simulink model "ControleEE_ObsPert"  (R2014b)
settings: Solver=ode45  StartTime=0.0  StopTime=60  RelTol=1e-6
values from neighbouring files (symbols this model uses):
  K = acker(A,B,[p p])    [para2nl.m]    (also in para2nl_PI.m = acker(Aa,Ba,[p,p,p]); PrPara2nl_PI.m = acker(Aa,Ba,[p,p,p]); TestesEE.m = acker(A,B,[p,-.6-1.02i,-.6+1.02i]); TestesEEobsPert.m = acker(A,B,[p,-.6-1.0198i,-.6+1.0198i]))
  L = L'    [para2nl.m]    (also in para2nl_PI.m; PrPara2nl_PI.m; TestesEE.m; TestesEEcanalI.m)
  Lc = L(4)    [TestesEEobsPert.m]
  Ls1 = L(5)    [TestesEEobsPert.m]
  Ls2 = L(6)    [TestesEEobsPert.m]
  Nb = gf.den{1}(1,3)/gf.num{1}(1,3)    [para2nl.m]    (also in PrPara2nl_PI.m; TestesEE.m = gf.den{1}(1,4)/gf.num{1}(1,4); TestesEEcanalI.m = -Ki/(100*p); TestesEEobsPert.m = gf.den{1}(1,4)/gf.num{1}(1,4))
  w0 = .5    (= 0.5)    [TestesEEobsPert.m]

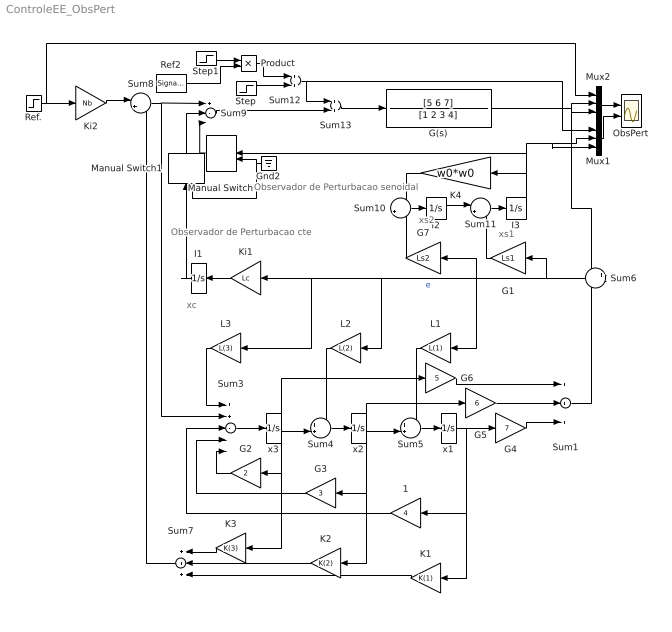
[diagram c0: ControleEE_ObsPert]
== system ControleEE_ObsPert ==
  note: xc
  note: xs1
  note: xs2
  note: Observador de Perturbacao cte
  note: Observador de Perturbacao senoidal
  1 : Gain  Gain=4
  G(s) : TransferFcn  Numerator=[5 6 7]  Denominator=[1 2 3 4]
  G1 : Gain  Gain=Ls1
  G2 : Gain  Gain=2
  G3 : Gain  Gain=3
  G4 : Gain  Gain=7
  G5 : Gain  Gain=6
  G6 : Gain  Gain=5
  G7 : Gain  Gain=Ls2
  Gnd2 : Ground
  I1 : Integrator
  I2 : Integrator
  I3 : Integrator
  K1 : Gain  Gain=K(1)
  K2 : Gain  Gain=K(2)
  K3 : Gain  Gain=K(3)
  K4 : Gain  Gain=w0*w0
  Ki1 : Gain  Gain=Lc
  Ki2 : Gain  Gain=Nb
  L1 : Gain  Gain=L(1)
  L2 : Gain  Gain=L(2)
  L3 : Gain  Gain=L(3)
  Manual Switch : ManualSwitch
  Manual Switch1 : ManualSwitch
  Mux1 : Mux  Inputs=3
  Mux2 : Mux  Inputs=3
  ObsPert : Scope  NumInputPorts=2
  Product : Product
  Ref. : Step  Time=0  SampleTime=0
  Ref2 : SignalGenerator  Amplitude=20  Frequency=w0  Units=rad/sec
  Step : Step  Time=3  After=3  SampleTime=0
  Step1 : Step  Time=2*pi/w0  SampleTime=0
  Sum1 : Sum  Inputs=+++
  Sum10 : Sum  Inputs=-+
  Sum11 : Sum  Inputs=|++
  Sum12 : Sum
  Sum13 : Sum
  Sum3 : Sum  Inputs=++---
  Sum4 : Sum  Inputs=++|
  Sum5 : Sum  Inputs=++|
  Sum6 : Sum  Inputs=+-
  Sum7 : Sum  Inputs=+++
  Sum8 : Sum  Inputs=|+-
  Sum9 : Sum  Inputs=+--
  x1 : Integrator
  x2 : Integrator
  x3 : Integrator
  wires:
  Ref./1 -> Mux2/1, Ki2/1
  Mux2/1 -> ObsPert/1
  x3/1 -> G6/1, Sum4/2, G2/1, K3/1
  x2/1 -> G5/1, Sum5/2, G3/1, K2/1
  Sum3/1 -> x3/1
  G2/1 -> Sum3/5
  G3/1 -> Sum3/4
  x1/1 -> G4/1, 1/1, K1/1
  1/1 -> Sum3/3
  G4/1 -> Sum1/3
  G5/1 -> Sum1/2
  G6/1 -> Sum1/1
  G(s)/1 -> Mux2/3, Sum6/1, Mux2/2
  Sum1/1 -> Sum6/2
  Sum13/1 -> G(s)/1
  Sum4/1 -> x2/1
  Sum5/1 -> x1/1
  Sum6/1 -> G1/1, L1/1, L2/1, L3/1, Ki1/1, G7/1  "e"
  L3/1 -> Sum3/1
  L2/1 -> Sum4/1
  L1/1 -> Sum5/1
  K3/1 -> Sum7/1
  K2/1 -> Sum7/2
  K1/1 -> Sum7/3
  Sum8/1 -> Sum3/2, Sum9/1
  Ki2/1 -> Sum8/1
  Sum7/1 -> Sum8/2
  Sum10/1 -> I2/1
  Sum11/1 -> I3/1
  K4/1 -> Sum10/1
  I2/1 -> Sum11/1
  G1/1 -> Sum11/2
  G7/1 -> Sum10/2
  Gnd2/1 -> Manual Switch1/2, Manual Switch/2
  Sum9/1 -> Sum13/2
  Manual Switch/1 -> Sum9/3
  Mux1/1 -> ObsPert/2
  I3/1 -> Manual Switch/1, Mux1/3, Mux1/2, K4/1
  Step/1 -> Sum12/2
  Sum12/1 -> Sum13/1, Mux1/1
  Manual Switch1/1 -> Sum9/2
  I1/1 -> Manual Switch1/1
  Step1/1 -> Product/1
  Ref2/1 -> Product/2
  Product/1 -> Sum12/1
  Ki1/1 -> I1/1
